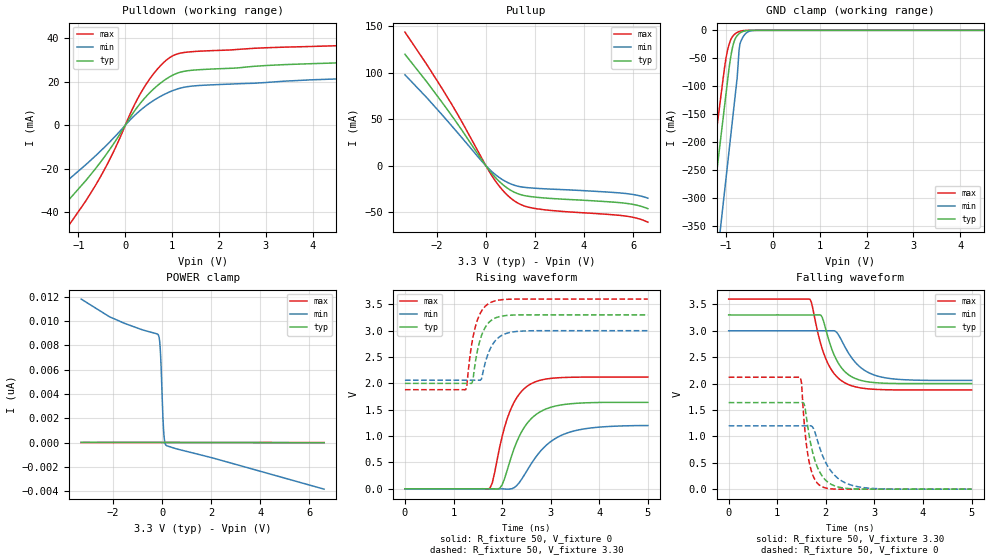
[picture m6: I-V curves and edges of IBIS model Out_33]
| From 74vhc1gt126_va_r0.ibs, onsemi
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|//////////////////////////////////////////////////////////////////////////////
|//////////////////////////////////////////////////////////////////////////////
[Model] Out_33
Model_type 3-state
Polarity Non-Inverting
Enable Active-High
Vmeas = 1.65
Vref = 3.30
Rref = 1k
Cref = 15pF
|  variable   typ   min   max
C_comp   3.8pF   3.8pF   3.8pF
|//////////////////////////////////////////////////////////////////////////////
[Temperature Range]   25   125   -55
|//////////////////////////////////////////////////////////////////////////////
[Voltage Range]   3.30V   3.00V   3.60V
|//////////////////////////////////////////////////////////////////////////////
[Pulldown Reference]   0V   0V   0V
|//////////////////////////////////////////////////////////////////////////////
[Pullup Reference]   3.30V   3.00V   3.60V
|//////////////////////////////////////////////////////////////////////////////
[GND Clamp Reference]   0V   0V   0V
|//////////////////////////////////////////////////////////////////////////////
[POWER Clamp Reference] 3.30V   3.00V   3.60V
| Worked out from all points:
|   slope of the pulldown table from 0 to 0.495 V, typ, clamps not added: 34.5 ohm
|   slope of the pullup table from 0 to 0.495 V, typ, clamps not added: 31.7 ohm
|   GND clamp passes 1 mA (typ) near -0.59 V on its own axis
|   falling waveform, R_fixture 50, V_fixture 3.30: 20-80 % time 362ps typ, 475ps min, 374ps max; typ from 3.3 V to 2 V
|   falling waveform, R_fixture 50, V_fixture 0: 20-80 % time 264ps typ, 391ps min, 158ps max; typ from 1.64 V to 0 V
|   rising waveform, R_fixture 50, V_fixture 0: 20-80 % time 484ps typ, 664ps min, 409ps max; typ from 0 V to 1.64 V
|   rising waveform, R_fixture 50, V_fixture 3.30: 20-80 % time 212ps typ, 248ps min, 212ps max; typ from 2 V to 3.3 V
|//////////////////////////////////////////////////////////////////////////////
[Pulldown]
|   Voltage   I(typ)   I(min)   I(max)
-3.6V     -124mA     -58.59mA   -149.4mA
-2.52V    -79.91mA   -43.55mA   -101.3mA
-1.68V    -46.59mA   -32.85mA   -63.16mA
-1.18V    -33.68mA   -24.42mA   -45.29mA
-440mV    -14.4mA    -10.03mA   -20.2mA
160mV     5.423mA    3.665mA    7.818mA
400mV     12.12mA    8.241mA    17.34mA
760mV     19.5mA     13.36mA    27.56mA
1.08V     23.68mA    16.43mA    32.55mA
3V        27.44mA    19.64mA    35.6mA
5.68V     29.78mA    22.31mA    37.93mA
7.2V      35.15mA    26.16mA    45.29mA
|//////////////////////////////////////////////////////////////////////////////
[Pullup]
|   Voltage   I(typ)   I(min)   I(max)
-3.3V     120mA      97.93mA    143.8mA
-2.42V    90.62mA    73.55mA    109.4mA
-1.4V     54.14mA    43.11mA    66.44mA
120mV     -4.264mA   -3.231mA   -5.499mA
560mV     -17.27mA   -12.96mA   -22.48mA
1.04V     -26.85mA   -19.85mA   -35.46mA
1.44V     -31.31mA   -22.76mA   -42mA
1.96V     -33.65mA   -24.14mA   -45.82mA
2.6V      -35.13mA   -25.12mA   -48.01mA
5.64V     -40.24mA   -29.73mA   -53.97mA
6.12V     -42.27mA   -31.52mA   -56.24mA
6.6V      -46.21mA   -34.89mA   -60.76mA
|//////////////////////////////////////////////////////////////////////////////
[GND Clamp]
|   Voltage   I(typ)   I(min)   I(max)
-3.3V     -1.735A    -2.002A    -1.552A
-1.48V    -453.2mA   -628.4mA   -361.6mA
-1.36V    -368.6mA   -537.8mA   -283.1mA
-1.28V    -312.3mA   -477.4mA   -230.8mA
-1.12V    -199.6mA   -356.6mA   -126.1mA
-1V       -115mA     -266mA     -50.64mA
-880mV    -39.3mA    -175.5mA   -13.96mA
-760mV    -9.466mA   -84.87mA   -3.902mA
-720mV    -6.073mA   -35.91mA   -2.358mA
-600mV    -1.174mA   -7.663mA   -256.9uA
-400mV    -11.43uA   -261.4uA   -196.1nA
6.6V      21.17pA    1.767nA    349.3fA
|//////////////////////////////////////////////////////////////////////////////
[POWER Clamp]
|   Voltage   I(typ)   I(min)   I(max)
-3.3V     21.17pA    11.8nA     360.7fA
-2.14V    17.02pA    10.34nA    316.7fA
-160mV    9.937pA    8.869nA    241.8fA
-120mV    9.794pA    8.609nA    240.2fA
-80mV     9.65pA     7.788nA    238.7fA
-60mV     9.579pA    7.052nA    238fA
-40mV     9.507pA    6.095nA    237.2fA
20mV      9.293pA    2.678nA    234.9fA
60mV      9.149pA    971.4pA    233.4fA
100mV     9.006pA    117.6pA    231.9fA
160mV     8.792pA    -226.9pA   229.6fA
6.6V      -14.26pA   -3.837nA   -14.23fA
|//////////////////////////////////////////////////////////////////////////////
|//////////////////////////////////////////////////////////////////////////////
[Ramp]
|  variable   typ   min   max
dV/dt_f   7.800E-01/3.750E-10  5.640E-01/4.750E-10  1.032E+00/3.750E-10
dV/dt_r   9.840E-01/5.000E-10  7.200E-01/7.000E-10  1.272E+00/4.000E-10
R_load = 50
|/////////////////////////////////////////////////////////////////////////////
[Falling Waveform]
R_fixture = 50
V_fixture = 3.30
V_fixture_min = 3.00
V_fixture_max = 3.60
C_fixture = 0p
|   time   V(typ)   V(min)   V(max)
0s        3.3V       3V         3.6V
1.675ns   3.3V       3V         3.595V
1.725ns   3.3V       3V         3.452V
1.9ns     3.293V     3V         2.735V
2.025ns   2.939V     3.001V     2.415V
2.225ns   2.439V     2.968V     2.131V
2.5ns     2.147V     2.53V      1.969V
2.8ns     2.044V     2.249V     1.907V
3.2ns     2.007V     2.113V     1.884V
5ns       2V         2.06V      1.88V
|//////////////////////////////////////////////////////////////////////////////
[Falling Waveform]
R_fixture = 50
V_fixture = 0
C_fixture = 0p
|   time   V(typ)   V(min)   V(max)
0s        1.64V      1.2V       2.12V
1.475ns   1.64V      1.2V       2.121V
1.5ns     1.64V      1.2V       2.011V
1.55ns    1.625V     1.2V       1.31V
1.65ns    1.053V     1.2V       544mV
1.775ns   545.7mV    1.081V     179.3mV
1.925ns   247.5mV    653.9mV    45.05mV
2.2ns     56.43mV    245.4mV    1.175mV
2.6ns     4.113mV    57.78mV    0V
5ns       0V         0V         0V
|//////////////////////////////////////////////////////////////////////////////
[Rising Waveform]
R_fixture = 50
V_fixture = 0
C_fixture = 0p
|   time   V(typ)   V(min)   V(max)
0s        0V         0V         0V
1.75ns    949.4uV    47.02uV    10.52mV
1.8ns     366.4uV    48.36uV    118.2mV
1.95ns    8.635mV    808.8uV    788mV
2.15ns    490.5mV    -6.431mV   1.446V
2.4ns     1.079V     178.1mV    1.849V
2.65ns    1.373V     544.7mV    2.017V
3ns       1.546V     894.9mV    2.094V
3.4ns     1.613V     1.077V     2.115V
5ns       1.64V      1.2V       2.12V
|//////////////////////////////////////////////////////////////////////////////
[Rising Waveform]
R_fixture = 50
V_fixture = 3.30
V_fixture_min = 3.00
V_fixture_max = 3.60
C_fixture = 0p
|   time   V(typ)   V(min)   V(max)
0s        2V         2.06V      1.88V
1.25ns    2V         2.06V      1.88V
1.275ns   2V         2.06V      1.961V
1.375ns   1.999V     2.06V      2.745V
1.475ns   2.54V      2.06V      3.155V
1.575ns   2.904V     2.082V     3.37V
1.675ns   3.095V     2.462V     3.482V
1.8ns     3.211V     2.733V     3.549V
2.325ns   3.299V     2.987V     3.6V
5ns       3.3V       3V         3.6V
